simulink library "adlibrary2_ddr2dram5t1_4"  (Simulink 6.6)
undefined symbols (not defined in the file or in its folder): Bit, Location, Lower, Width
libraries: xbsIndex_r4 x26, adlibrary2_ddr2dram5t1_1 x1

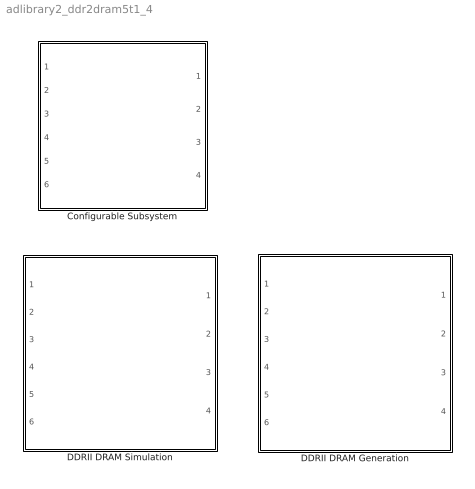
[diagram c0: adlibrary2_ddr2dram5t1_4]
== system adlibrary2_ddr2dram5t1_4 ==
  Configurable Subsystem : Subsystem  BlockChoice=DDRII DRAM Simulation
  DDRII DRAM Generation : Subsystem
  DDRII DRAM Simulation : Subsystem

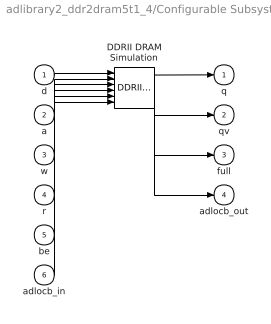
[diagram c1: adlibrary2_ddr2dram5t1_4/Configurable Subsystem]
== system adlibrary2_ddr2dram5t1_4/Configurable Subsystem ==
  d : Inport
  a : Inport  Port=2
  w : Inport  Port=3
  r : Inport  Port=4
  be : Inport  Port=5
  adlocb_in : Inport  Port=6
  DDRII DRAM Simulation : adlibrary2_ddr2dram5t1_1/DDRII DRAM Simulation  SystemSampleTime=-1
  q : Outport
  qv : Outport  Port=2
  full : Outport  Port=3
  adlocb_out : Outport  Port=4
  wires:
  d/1 -> DDRII DRAM Simulation/1
  a/1 -> DDRII DRAM Simulation/2
  w/1 -> DDRII DRAM Simulation/3
  r/1 -> DDRII DRAM Simulation/4
  be/1 -> DDRII DRAM Simulation/5
  adlocb_in/1 -> DDRII DRAM Simulation/6
  DDRII DRAM Simulation/1 -> q/1
  DDRII DRAM Simulation/2 -> qv/1
  DDRII DRAM Simulation/3 -> full/1
  DDRII DRAM Simulation/4 -> adlocb_out/1

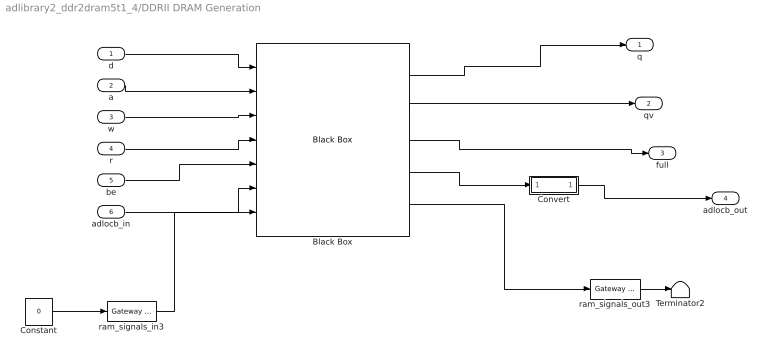
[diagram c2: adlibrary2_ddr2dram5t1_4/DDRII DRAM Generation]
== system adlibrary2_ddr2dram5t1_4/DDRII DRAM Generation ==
  d : Inport
  a : Inport  Port=2
  w : Inport  Port=3
  r : Inport  Port=4
  be : Inport  Port=5
  adlocb_in : Inport  Port=6
  Black Box : xbsIndex_r4/Black Box  init_code=ddr2sdram_v5_config3  sim_method=Inactive  block_type=blackbox2
  Constant : Constant  Value=0
  Convert : Subsystem
  Terminator2 : Terminator
  ram_signals_in3 : xbsIndex_r4/Gateway In  arith_type=Unsigned  n_bits=133  bin_pt=0  quantization="Round  (unbiased: +/- Inf)"  overflow=Saturate  period=ad_get_simulink_period  dbl_ovrd=off  timing_constraint=None  locs_specified=off  LOCs={}  block_type=gatewayin
  ram_signals_out3 : xbsIndex_r4/Gateway Out  hdl_port=on  timing_constraint=None  locs_specified=off  LOCs={}  block_type=gatewayout
  q : Outport
  qv : Outport  Port=2
  full : Outport  Port=3
  adlocb_out : Outport  Port=4
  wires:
  ram_signals_out3/1 -> Terminator2/1
  Constant/1 -> ram_signals_in3/1
  d/1 -> Black Box/1
  a/1 -> Black Box/2
  w/1 -> Black Box/3
  r/1 -> Black Box/4
  be/1 -> Black Box/5
  adlocb_in/1 -> Black Box/6
  Black Box/1 -> q/1
  Black Box/2 -> qv/1
  Black Box/3 -> full/1
  Black Box/4 -> Convert/1(in0)
  Convert/1(out0) -> adlocb_out/1
  ram_signals_in3/1 -> Black Box/7
  Black Box/5 -> ram_signals_out3/1

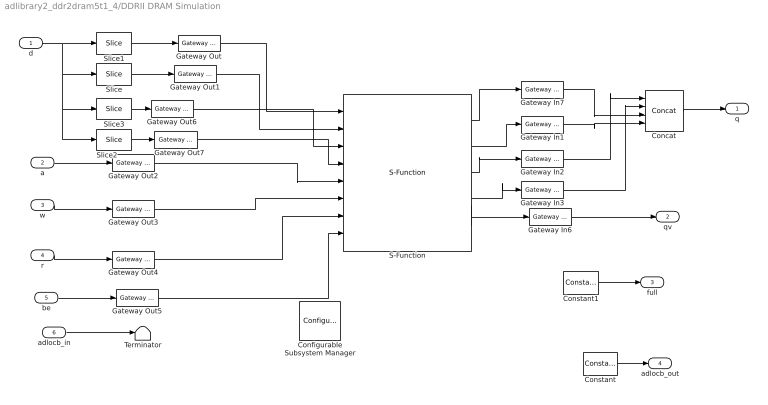
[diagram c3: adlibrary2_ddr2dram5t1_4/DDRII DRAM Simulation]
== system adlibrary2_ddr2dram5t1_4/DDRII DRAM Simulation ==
  d : Inport
  a : Inport  Port=2
  w : Inport  Port=3
  r : Inport  Port=4
  be : Inport  Port=5
  adlocb_in : Inport  Port=6
  Concat : xbsIndex_r4/Concat  num_inputs=4  dbl_ovrd=off  block_type=concat
  Configurable Subsystem Manager : xbsIndex_r4/Configurable Subsystem Manager  Tag=xcfgMgr  block_type=configsubsys
  Constant : xbsIndex_r4/Constant  arith_type=Signed (2's comp)  const=0  n_bits=66  bin_pt=0  explicit_period=on  period=ad_get_simulink_period  equ=P=C  opselect=C  inp2=PCIN>>17  opr=+  inp1=P  carry=CIN  dbl_ovrd=off  block_type=constant
  Constant1 : xbsIndex_r4/Constant  arith_type=Boolean  const=0  n_bits=66  bin_pt=0  explicit_period=on  period=ad_get_simulink_period  equ=P=C  opselect=C  inp2=PCIN>>17  opr=+  inp1=P  carry=CIN  dbl_ovrd=off  block_type=constant
  Gateway In{1..3,7} (4 alike) : xbsIndex_r4/Gateway In  arith_type=Unsigned  n_bits=32  bin_pt=0  quantization="Round  (unbiased: +/- Inf)"  overflow=Saturate  period=ad_get_simulink_period  dbl_ovrd=on  timing_constraint=None  locs_specified=off  LOCs={}  block_type=gatewayin
  Gateway In6 : xbsIndex_r4/Gateway In  arith_type=Boolean  n_bits=1  bin_pt=0  quantization="Round  (unbiased: +/- Inf)"  overflow=Saturate  period=ad_get_simulink_period  dbl_ovrd=on  timing_constraint=None  locs_specified=off  LOCs={}  block_type=gatewayin
  Gateway Out{,1..7} (8 alike) : xbsIndex_r4/Gateway Out  hdl_port=off  timing_constraint=None  locs_specified=off  LOCs={}  block_type=gatewayout
  S-Function : S-Function  FunctionName=ddr2dram128  Parameters=3
  Slice : xbsIndex_r4/Slice  nbits=32  boolean_output=off  mode=Lower Bit Location + Width  bit1=0  base1=MSB of Input  bit0=0  base0=LSB of Input  dbl_ovrd=off  block_type=slice
  Slice1 : xbsIndex_r4/Slice  nbits=32  boolean_output=off  mode=Lower Bit Location + Width  bit1=0  base1=MSB of Input  bit0=32  base0=LSB of Input  dbl_ovrd=off  block_type=slice
  Slice2 : xbsIndex_r4/Slice  nbits=32  boolean_output=off  mode=Lower Bit Location + Width  bit1=0  base1=MSB of Input  bit0=64  base0=LSB of Input  dbl_ovrd=off  block_type=slice
  Slice3 : xbsIndex_r4/Slice  nbits=32  boolean_output=off  mode=Lower Bit Location + Width  bit1=0  base1=MSB of Input  bit0=96  base0=LSB of Input  dbl_ovrd=off  block_type=slice
  Terminator : Terminator
  q : Outport
  qv : Outport  Port=2
  full : Outport  Port=3
  adlocb_out : Outport  Port=4
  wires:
  Gateway In2/1 -> Concat/1
  Gateway In3/1 -> Concat/2
  Gateway In1/1 -> Concat/4
  Gateway In7/1 -> Concat/3
  Gateway Out5/1 -> S-Function/8
  Gateway Out4/1 -> S-Function/7
  Gateway Out3/1 -> S-Function/6
  Gateway Out2/1 -> S-Function/5
  Gateway Out7/1 -> S-Function/4
  Gateway Out6/1 -> S-Function/3
  Gateway Out1/1 -> S-Function/2
  Gateway Out/1 -> S-Function/1
  S-Function/4 -> Gateway In3/1
  S-Function/3 -> Gateway In2/1
  S-Function/2 -> Gateway In1/1
  S-Function/1 -> Gateway In7/1
  S-Function/5 -> Gateway In6/1
  Slice2/1 -> Gateway Out7/1
  Slice3/1 -> Gateway Out6/1
  Constant1/1 -> full/1
  adlocb_in/1 -> Terminator/1
  Constant/1 -> adlocb_out/1
  a/1 -> Gateway Out2/1
  w/1 -> Gateway Out3/1
  r/1 -> Gateway Out4/1
  Gateway In6/1 -> qv/1
  be/1 -> Gateway Out5/1
  Slice1/1 -> Gateway Out/1
  Slice/1 -> Gateway Out1/1
  d/1 -> Slice3/1, Slice2/1, Slice/1, Slice1/1
  Concat/1 -> q/1

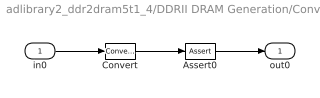
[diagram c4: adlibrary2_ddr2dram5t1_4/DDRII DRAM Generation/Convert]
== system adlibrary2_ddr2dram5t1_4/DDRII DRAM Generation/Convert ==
  in0 : Inport
  Assert0 : xbsIndex_r4/Assert  assert_type=off  type_source=Explicitly  arith_type="Signed  (2's comp)"  n_bits=16  bin_pt=14  assert_rate=on  rate_source=Explicitly  period=ad_get_simulink_period  output_port=on  block_type=assert
  Convert : xbsIndex_r4/Convert  arith_type=Unsigned  n_bits=66  bin_pt=0  quantization=Truncate  overflow=Wrap  latency=0  dbl_ovrd=off  pipeline=off  block_type=convert
  out0 : Outport
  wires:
  in0/1 -> Convert/1
  Convert/1 -> Assert0/1
  Assert0/1 -> out0/1
